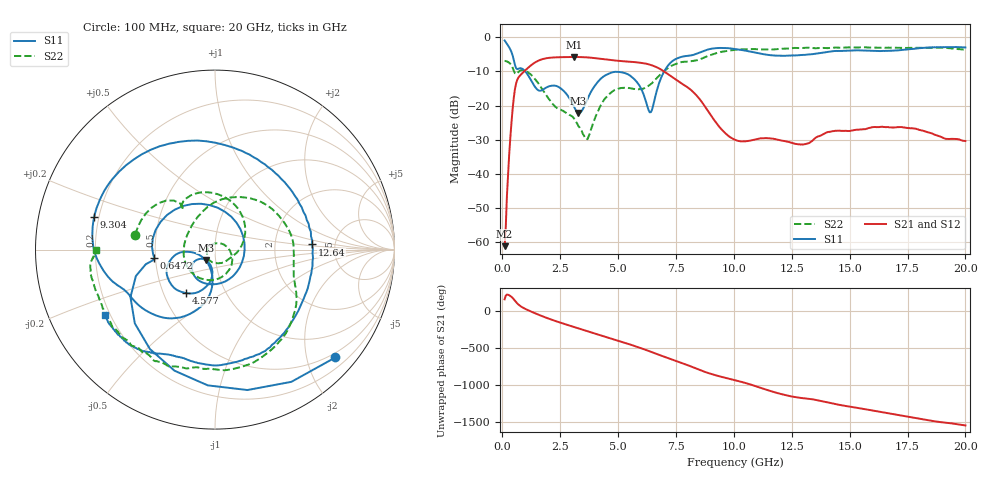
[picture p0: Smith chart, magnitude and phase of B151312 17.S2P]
!  2-Port S-parameters saved by WinCal
! VAR MeasName=S-Parameters (CALIBRATED_DATA) read from VNA (N5244A)
! VAR MeasDate=12/8/2015 5:44:49 PM
! VAR NAME=B151312 17
! VAR FILENAME=B151312 17.S2P
! VAR DATE=12/8/2015 5:44:49 PM
! VAR PHYS_PORTS=1,2
# Hz S DB R 50
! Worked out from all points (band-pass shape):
!   401 points, 100 MHz to 20 GHz, reference 50 ohm
!   highest |S21| = -5.74 dB at 3.085 GHz (marker M1); lowest = -61.3 dB at 100 MHz (marker M2)
!   |S21| within 3 dB of the highest: 1.147 GHz to 6.657 GHz (5.511 GHz wide, 141 % of centre)
!   lowest |S11| = -22.2 dB at 3.284 GHz (marker M3), VSWR 1.17, Z = 44.8 - j5.26 ohm
!   |S11| at or under -10 dB: 995.2 MHz to 6.991 GHz (5.996 GHz wide, 150 % of centre)
!   |S22| runs from -29.9 to -2.9 dB; largest |S21 - S12| = 0.0016
!   S11 on the Smith chart (normalised r, x): 100 MHz: 0.40, -2.56; 647.2 MHz: 0.49, -0.05; 4.577 GHz: 0.65, -0.34; 9.304 GHz: 0.18, +0.13; 12.64 GHz: 3.34, +0.27; 20 GHz: 0.18, -0.27
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1e8  -0.91 -41.9  -61.28 156.3  -60.70 160.3  -6.90 169.3
3.985e8  -4.34 -137.4  -24.84 -170.0  -24.83 -170.0  -8.26 135.1
6.4725e8  -9.33 -171.9  -12.44 100.6  -12.44 100.6  -10.53 129.4
1.294e9  -13.24 75.2  -7.93 -16.5  -7.93 -16.5  -11.33 65.5
1.94075e9  -14.58 -72.6  -6.08 -98.2  -6.08 -98.2  -17.38 -0.0
2.53775e9  -15.05 -134.6  -5.82 -162.8  -5.82 -162.8  -21.28 -54.3
3.085e9  -20.22 -148.2  -5.74 142.3  -5.75 142.3  -23.70 -120.1
3.284e9  -22.21 -131.3  -5.77 122.5  -5.76 122.5  -26.01 -152.1
3.43325e9  -21.58 -112.0  -5.80 107.8  -5.79 107.8  -27.51 175.7
4.5775e9  -10.71 -123.9  -6.58 -3.7  -6.57 -3.7  -16.96 -60.3
5.5725e9  -11.51 -164.6  -7.17 -101.3  -7.18 -101.4  -15.01 -165.6
6.3685e9  -22.01 -143.0  -8.01 171.4  -8.00 171.4  -14.01 121.9
6.7665e9  -13.52 -94.6  -9.10 124.6  -9.10 124.6  -11.33 86.9
7.662e9  -5.88 -136.9  -13.16 23.6  -13.12 23.4  -7.38 13.7
9.30375e9  -3.13 165.0  -25.67 -161.0  -25.67 -161.2  -4.52 -45.5
1.005e10  -3.40 131.8  -30.06 139.7  -30.12 139.2  -3.66 -67.4
1.119425e10  -4.85 77.1  -29.62 32.9  -29.69 32.9  -3.55 -92.5
1.2637e10  -5.33 3.1  -31.22 -88.0  -31.25 -87.6  -3.10 -111.6
1.338325e10  -4.94 -30.7  -30.42 -118.1  -30.36 -117.5  -3.15 -121.1
1.4627e10  -3.98 -73.6  -27.45 161.9  -27.38 162.0  -3.05 -133.6
1.67165e10  -3.96 -111.5  -26.42 49.0  -26.25 49.0  -3.03 -152.4
2e10  -2.96 -149.2  -30.43 -113.3  -30.48 -114.6  -3.61 -179.9
